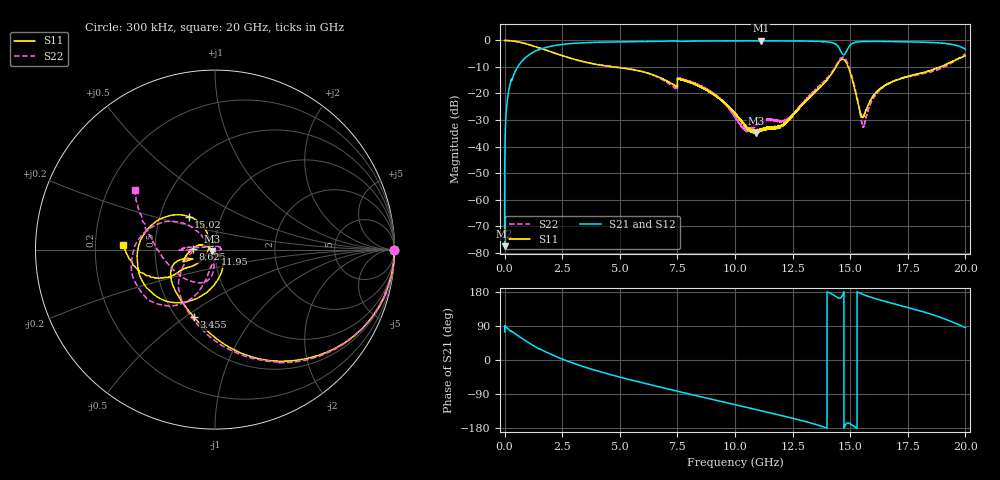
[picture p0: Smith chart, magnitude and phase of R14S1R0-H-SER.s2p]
!{R14S1R0}
!Johanson Technology Inc.
!www.johansontechnology.com
!Test Board Conditions:
!Substrate Type  RO4350B
!Substrate Thickness  20 mil
!Substrate Dk  3.66
!TL Type: GCPW
!TL Trace Width  36 mil
!TL Gap  12 mil
!Electrode orientation  Horizontal
!DUT TOPOLOGY	SERIES
!Mounting Pad LxW  26x36 mil
! Created Wed Nov 25 17:33:21 2020
! 2 Port Network Data from SP1.SP block
! freq  magS11  angS11  magS21  angS21  magS12  angS12  magS22  angS22
# khz S ma R 50
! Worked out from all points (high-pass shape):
!   20001 points, 300 kHz to 20 GHz, reference 50 ohm
!   highest |S21| = -0.13 dB at 11.12 GHz (marker M1); lowest = -77.6 dB at 300 kHz (marker M2)
!   |S21| within 3 dB of the highest: 1.616 GHz to 14.54 GHz (12.92 GHz wide, 160 % of centre); 14.9 GHz to 19.97 GHz (5.07 GHz wide, 29.1 % of centre)
!   lowest |S11| = -34.9 dB at 10.93 GHz (marker M3), VSWR 1.04, Z = 48.5 - j1.01 ohm
!   |S11| at or under -10 dB: 4.735172 GHz to 4.737514 GHz (2.342 MHz wide, 0.0494 % of centre); 4.738 GHz to 14.38 GHz (9.642 GHz wide, 101 % of centre); 14.92 GHz to 18.9 GHz (3.986 GHz wide, 23.6 % of centre)
!   |S22| runs from -34.5 to 0.0 dB; largest |S21 - S12| = 0.014
!   S11 on the Smith chart (normalised r, x): 300 kHz: open; 3.455 GHz: 0.61, -0.54; 8.625 GHz: 0.78, +0.01; 11.95 GHz: 1.00, -0.05; 15.02 GHz: 0.70, +0.27; 20 GHz: 0.32, +0.02
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300  0.9972 -0.2  0.000132 74.3  0.0002257 75.4  0.997 -0.2
101300  0.9977 -4.9  0.06462 84.7  0.06495 84.8  0.9972 -4.9
131300  0.9954 -6.3  0.08355 83.3  0.0839 83.4  0.9963 -6.4
506300  0.9564 -22.2  0.2855 67.2  0.2859 67.4  0.9558 -22.3
1422300  0.7394 -57.2  0.6552 31.9  0.6557 31.9  0.743 -57.9
3334300  0.4053 -104.8  0.8994 -15.7  0.8997 -15.7  0.4065 -107.3
3455300  0.3934 -107.5  0.9047 -18.1  0.9047 -18.1  0.3951 -109.5
6667300  0.2061 -163.6  0.9665 -70.2  0.9666 -70.1  0.2006 -152.3
8625300  0.1253 177.8  0.9759 -98.5  0.9768 -98.5  0.1314 174.7
1.00003e7  0.04222 157.0  0.9817 -117.9  0.9822 -117.9  0.0363 149.7
1.09323e7  0.01793 -144.7  0.9824 -131.0  0.9794 -131.1  0.02518 45.2
1.11183e7  0.02089 -133.6  0.9852 -133.8  0.9809 -133.7  0.0302 29.6
1.19483e7  0.02349 -87.0  0.9798 -145.8  0.9804 -145.6  0.03013 -19.2
1.33343e7  0.093 -61.8  0.9672 -167.1  0.9695 -167.0  0.09966 -102.8
1.44613e7  0.3653 -125.8  0.7871 164.4  0.7895 164.4  0.3887 -126.4
1.47153e7  0.4351 -175.7  0.5355 178.0  0.5348 177.9  0.4766 -167.9
1.50173e7  0.2348 128.6  0.8278 -168.9  0.825 -168.9  0.2573 143.2
1.55703e7  0.03693 178.3  0.9571 172.6  0.9563 172.6  0.02357 -156.7
1.60243e7  0.09321 -141.9  0.9611 163.3  0.9623 163.4  0.08411 -93.7
1.66673e7  0.1535 -144.1  0.956 152.1  0.9523 152.2  0.1539 -98.6
1.85103e7  0.2724 -148.3  0.9168 121.0  0.9141 120.8  0.2567 -152.8
2e7  0.5148 176.9  0.6827 85.4  0.6718 85.5  0.5568 142.9
